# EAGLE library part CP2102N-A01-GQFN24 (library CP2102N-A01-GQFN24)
SILICON LABS - CP2102N-A01-GQFN24 - USB-UART INTERFACE BRIDGE, QFN-24 Source: Datasheet
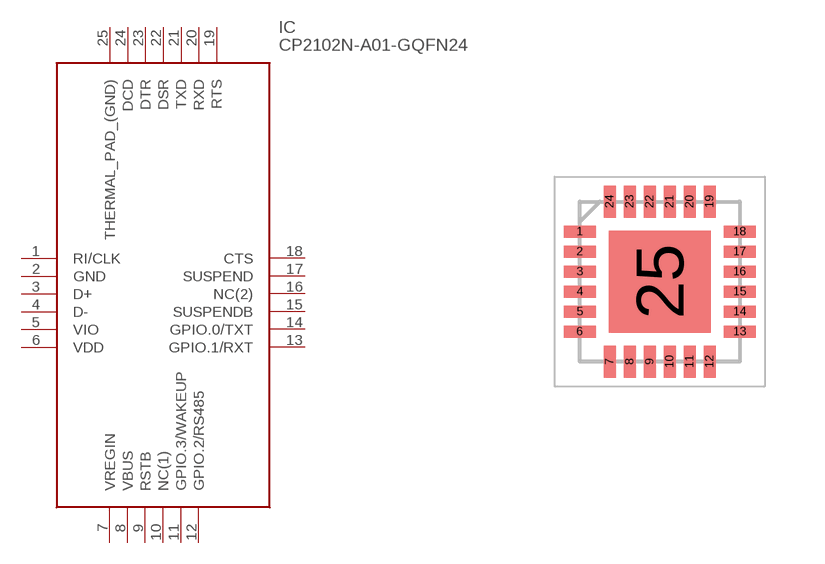
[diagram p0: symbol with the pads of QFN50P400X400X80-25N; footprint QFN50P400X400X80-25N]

Designator prefix IC

## CP2102N-A01-GQFN24 (Arrow_Part_Number: CP2102N-A01-GQFN24; Arrow_Price/Stock: https://www.arrow.com/en/products/cp2102n-a01-gqfn24/silicon-labs; Description: SILICON LABS - CP2102N-A01-GQFN24 - USB-UART INTERFACE BRIDGE, QFN-24; Height: 0.8mm; Manufacturer_Name: Silicon Labs; Manufacturer_Part_Number: CP2102N-A01-GQFN24)  [QFN50P400X400X80-25N]
1  RI/CLK
2  GND
3  D+
4  D-
5  VIO
6  VDD
7  VREGIN
8  VBUS
9  RSTB
10  NC(1)  nc
11  GPIO.3/WAKEUP
12  GPIO.2/RS485
13  GPIO.1/RXT
14  GPIO.0/TXT
15  SUSPENDB
16  NC(2)  nc
17  SUSPEND
18  CTS
19  RTS
20  RXD
21  TXD
22  DSR
23  DTR
24  DCD
25  THERMAL_PAD_(GND)

## Footprint QFN50P400X400X80-25N (pad centres in mm)
QFN-24 (4x4 mm)_1
smd 0.8 x 0.3: 1 -2,1.25; 2 -2,0.75; 3 -2,0.25; 4 -2,-0.25; 5 -2,-0.75; 6 -2,-1.25; 13 2,-1.25; 14 2,-0.75; 15 2,-0.25; 16 2,0.25; 17 2,0.75; 18 2,1.25
smd 0.3 x 0.8: 7 -1.25,-2; 8 -0.75,-2; 9 -0.25,-2; 10 0.25,-2; 11 0.75,-2; 12 1.25,-2; 19 1.25,2; 20 0.75,2; 21 0.25,2; 22 -0.25,2; 23 -0.75,2; 24 -1.25,2
smd 2.55 x 2.55: 25 0,0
